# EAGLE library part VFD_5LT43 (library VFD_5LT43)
Futaba 5LT43 VFD Filament: 2.7 - 3.3 Vac, 3.0V recommended Anode/Grid: 34Vp-p max, 26V recommended
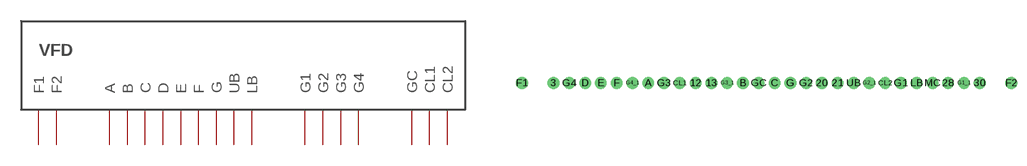
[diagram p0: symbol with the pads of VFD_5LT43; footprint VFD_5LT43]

Designator prefix -

## VFD_5LT43  [VFD_5LT43]
A  A
B  B
C  C
CL1  CL1
CL2  CL2
D  D
E  E
F  F
F1  F1
F2  F2
G  G
G1  G1
G2  G2
G3  G3
G4  G4
GC  GC
LB  LB
UB  UB

## Footprint VFD_5LT43 (pad centres in mm)
drill 1.016 pad 1.88: 3 7.62,0; 12 30.48,0; 13 33.02,0; 20 50.8,0; 21 53.34,0; 28 71.12,0; 30 76.2,0; A 22.86,0; B 38.1,0; C 43.18,0; CL1 27.94,0; CL2 60.96,0; D 12.7,0; E 15.24,0; F 17.78,0; F1 2.54,0; F2 81.28,0; G 45.72,0; G1 63.5,0; G1_1 73.66,0; G2 48.26,0; G2_1 58.42,0; G3 25.4,0; G3_1 35.56,0; G4 10.16,0; G4_1 20.32,0; GC 40.64,0; LB 66.04,0; MC 68.58,0; UB 55.88,0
